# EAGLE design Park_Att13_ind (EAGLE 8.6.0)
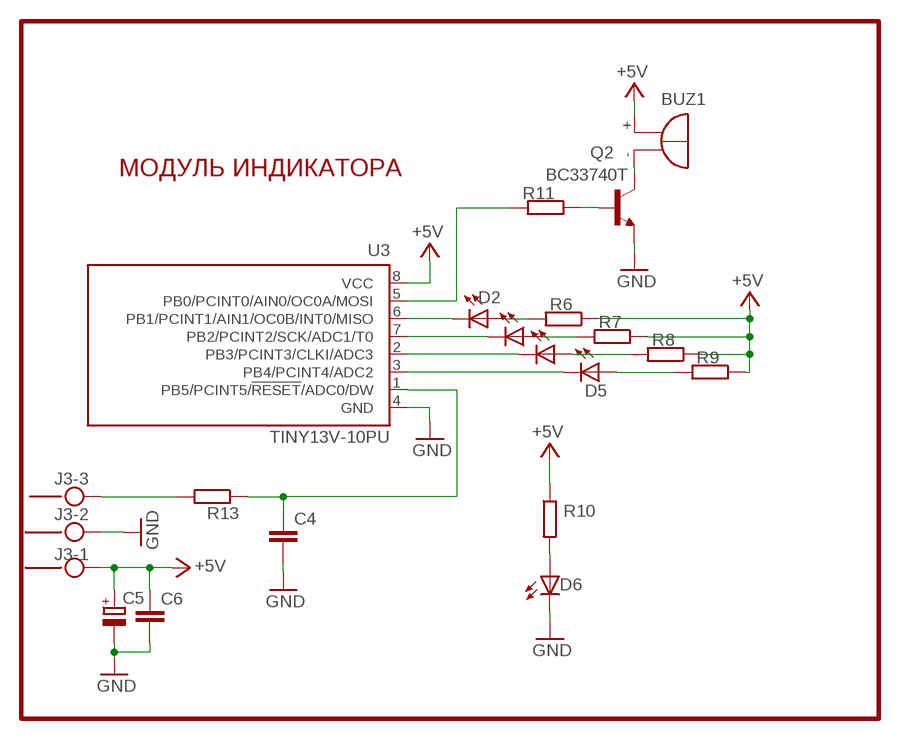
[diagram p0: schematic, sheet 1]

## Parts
BUZ1  F/HMB  [F/HMB]
C4  C-EUC1206  [C1206]
C5  CPOL-EUC/6032-28W  [C/6032-28W]
C6  C-EUC1206  [C1206]
D2  LED5MM  [LED5MM]
D3  LED5MM  [LED5MM]
D4  LED5MM  [LED5MM]
D5  LED5MM  [LED5MM]
D6  LED5MM  [LED5MM]
J3  MKDSN1,5/3-5,08  [MKDSN1,5/3-5,08]
Q2  BC33740T  BC337  [TO92]
R6  R-EU_R1206  [R1206]
R7  R-EU_R1206  [R1206]
R8  R-EU_R1206  [R1206]
R9  R-EU_R1206  [R1206]
R10  R-EU_R1206  [R1206]
R11  R-EU_R1206  [R1206]
R13  R-EU_R1206  [R1206]
U3  TINY13V-10PU  [DIL08]

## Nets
+5V: BUZ1.+ C5.+ C6.1 J3.1 R6.1 R7.1 R8.1 R9.1 R10.1 U3.8(VCC)
GND: C4.2 C5.- C6.2 D6.K(C) J3.2 Q2.1(E) U3.4(GND)
N$4: J3.3 R13.2
N$5: C4.1 R13.1 U3.1(PB5/PCINT5/!RESET!/ADC0/DW)
N$6: D2.K(C) U3.6(PB1/PCINT1/AIN1/OC0B/INT0/MISO)
N$7: D3.K(C) U3.7(PB2/PCINT2/SCK/ADC1/T0)
N$8: D4.K(C) U3.2(PB3/PCINT3/CLKI/ADC3)
N$9: D5.K(C) U3.3(PB4/PCINT4/ADC2)
N$10: R11.2 U3.5(PB0/PCINT0/AIN0/OC0A/MOSI)
N$11: D6.A R10.2
N$12: D3.A R7.2
N$13: D4.A R8.2
N$14: D5.A R9.2
N$17: D2.A R6.2
N$21: Q2.2(B) R11.1
N$22: BUZ1.- Q2.3(C)

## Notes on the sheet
- МОДУЛЬ ИНДИКАТОРА

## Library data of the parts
BUZ1 = buzzer:F/HMB: BUZZER; OC_FARNELL: unknown; OC_NEWARK: unknown
C4 C6 = rcl:C-EU: CAPACITOR, European symbol
C5 = rcl:CPOL-EU: POLARIZED CAPACITOR, European symbol
D2-D6 = led:LED: LED
J3 = con-phoenix-508:MKDSN1,5/3-5,08: MKDSN 1,5/ 3-5,08 Printklemme Nennstrom: 13,5 A Nennspannung: 250 V Rastermaß: 5,08 mm Polzahl: 3 Anschlussart: Schraubanschluss Montage: Löten Anschlussrichtung Leiter/Platine: 0 ° Artikelnummer: 1729131 Source: http://eshop.phoenixcontact.com .. 1729131.pdf
Q2 = transistor:BC337: NPN TRANSISTOR
R6-R11 R13 = rcl:R-EU_: RESISTOR, European symbol
U3 = atmel:TINY13: 8-bit AVR Microcontroller with 1K Bytes In-System Programmable Flash Source: http://www.atmel.com/dyn/resources/prod_documents/2535S.pdf; MPN: ATTINY13V-10PU; OC_FARNELL: 9171576; OC_NEWARK: 96K6523

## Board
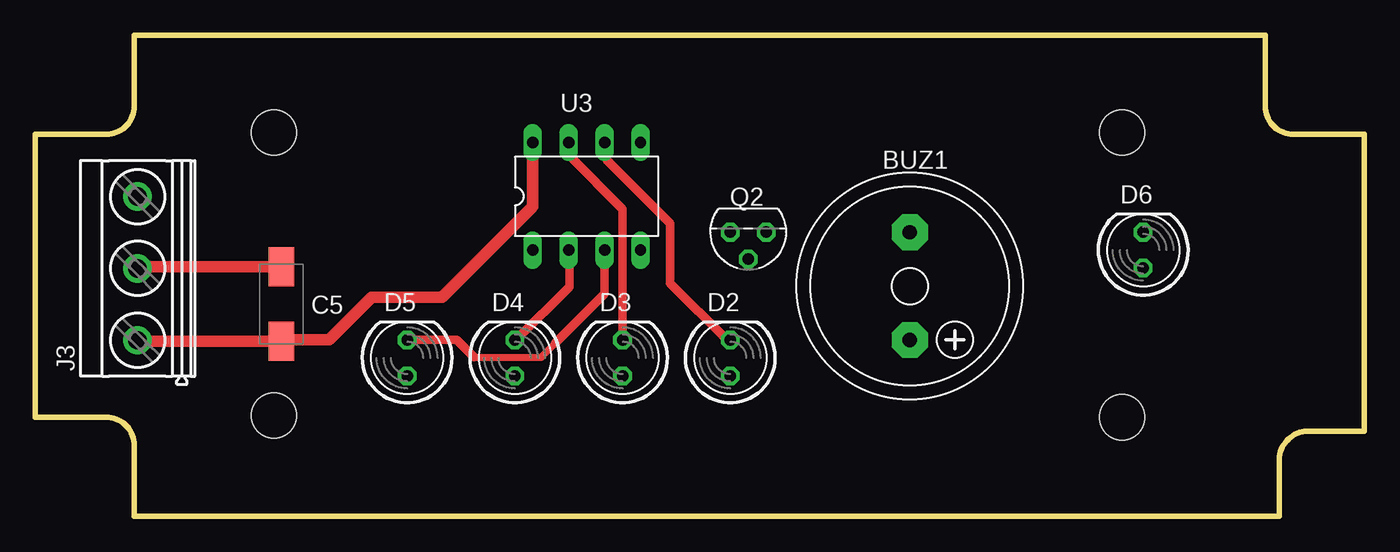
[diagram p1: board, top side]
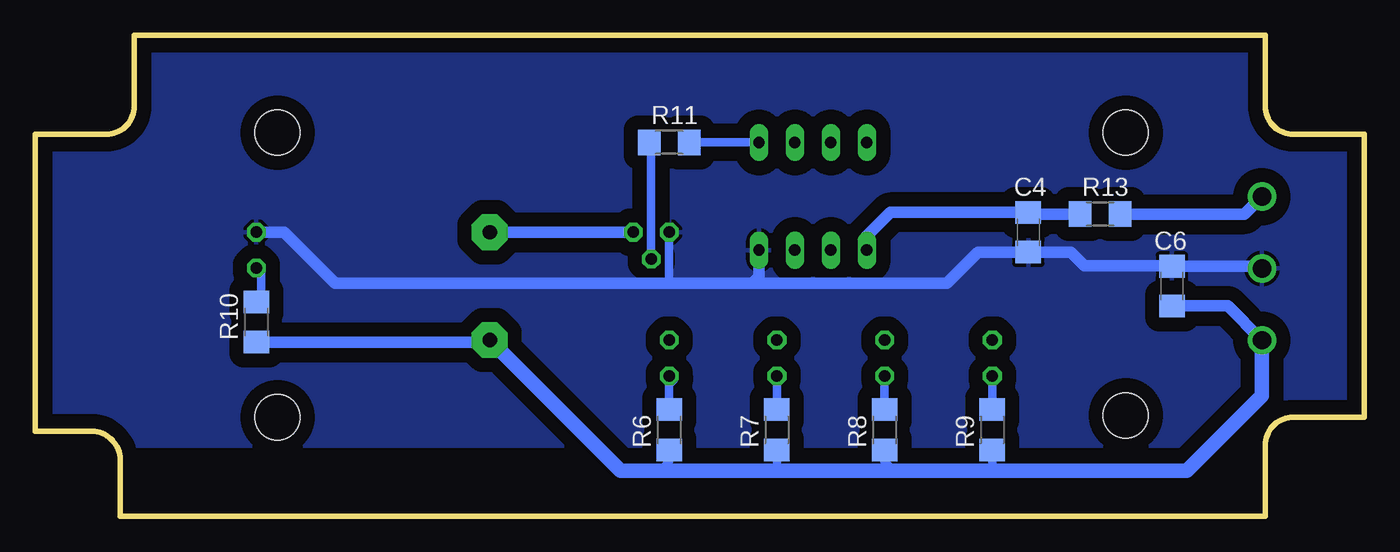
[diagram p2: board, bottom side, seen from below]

Size 94 x 34 mm. Coordinates in mm from the lower left corner, seen from the top.
Outline: 7,0 7,5 arc90 5,7 0,7 0,27 5,27 arc90 7,29 7,34 87,34 87,29 arc90 89,27 94,27 94,6 90,6 arc90 88,4 88,0 7,0
Copper layers (1*16): Top 0.035mm / dielectric 1.5mm / Bottom 0.035mm
Design rules "default": minimum track width 10mil, minimum drill 24mil, track to track 8mil, track to pad 8mil, pad to pad 8mil, via to via 8mil, smd to smd 8mil, copper to edge 40mil, drill to drill 8mil, minimum pad ring 10mil, minimum via ring 8mil, stop-mask expansion 4mil, vias tented up to drill 0mil, thermal gap 10mil
Holes 3.2 mm at 16.88,7.12 76.88,7 16.88,27.12 76.88,27.12

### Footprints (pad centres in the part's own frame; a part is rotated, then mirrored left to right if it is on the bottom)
F/HMB = drill 1.016 pad 2.54 octagon: + 3.81,0; - -3.81,0
C1206 = smd 1.6 x 1.8: 1 -1.4,0; 2 1.4,0
C/6032-28W = smd 2.75 x 1.8: + 2.625,0; - -2.625,0
LED5MM = drill 0.813 octagon: A -1.27,0; K 1.27,0
MKDSN1,5/3-5,08 = drill 1.3 pad 2: 1 -7.641,0.025; 2 -2.561,0.025; 3 2.519,0.025
TO92 = drill 0.813 octagon: 1 1.27,0; 2 0,1.905; 3 -1.27,0
R1206 = smd 1.6 x 1.803: 1 -1.422,0; 2 1.422,0
DIL08 = drill 0.813 long: 1 -3.81,-3.81; 2 -1.27,-3.81; 3 1.27,-3.81; 4 3.81,-3.81; 5 3.81,3.81; 6 1.27,3.81; 7 -1.27,3.81; 8 -3.81,3.81

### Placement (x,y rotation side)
BUZ1  61.86,16.27 270 top
C4  23.76,20.08 270 bottom
C5  17.41,15 270 top
C6  13.6,16.27 90 bottom
D2  49.16,11.19 90 top
D3  41.54,11.19 90 top
D4  33.92,11.19 90 top
D5  26.3,11.19 90 top
D6  78.37,18.81 90 top
J3  7.25,20.08 90 top
Q2  50.43,20.08 180 top
R6  49.16,6.11 90 bottom
R7  41.54,6.11 90 bottom
R8  33.92,6.11 90 bottom
R9  26.3,6.11 90 bottom
R10  78.37,13.73 90 bottom
R11  49.16,26.43 0 bottom
R13  18.68,21.35 0 bottom
U3  39,22.62 0 top

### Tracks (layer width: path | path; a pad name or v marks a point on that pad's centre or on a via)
+5V
  Top 0.813: U3.8 35.19,21.88 28.78,15.47 23.78,15.47 20.78,12.47 17.51,12.47 C5.+ 7.29,12.38 J3.1
  Bottom 0.61: R9.1 26.3,3.45 26.53,3.22 | R8.1 33.92,3.86 33.28,3.22 | R7.1 41.54,3.48 41.28,3.22 | R6.1 49.16,3.84 49.78,3.22
  Bottom 0.813: C6.1 9.66,14.87 J3.1 | R10.1 62.01,12.31 BUZ1.+
  Bottom 1.016: J3.1 7.23,8.53 12.53,3.22 26.53,3.22 33.28,3.22 41.28,3.22 49.78,3.22 52.62,3.22 BUZ1.+
GND
  Top 0.813: C5.- 7.33,17.62 J3.2
  Bottom 0.61: Q2.1 49.16,16.59 49.28,16.47
  Bottom 0.813: J3.2 7.38,17.67 C6.2 13.65,17.72 19.78,17.72 20.74,18.68 C4.2 27.32,18.68 29.53,16.47 43.28,16.47 | D6.K 76.39,20.08 72.78,16.47 49.28,16.47 43.28,16.47 | U3.4 42.81,16.94 43.28,16.47
  pour Bottom (isolate 1.016): 0.53,33.97 94.28,33.97 94.03,4.97 0.53,4.97
N$4
  Bottom 0.813: R13.2 8.47,21.35 J3.3
N$5
  Bottom 0.813: R13.1 23.63,21.35 C4.1 33.52,21.48 35.28,19.72 35.28,18.9 U3.1
N$6
  Top 0.61: D2.K 48.91,12.46 44.91,16.47 44.91,20.72 40.41,25.22 40.41,26.29 U3.6
N$7
  Top 0.61: D3.K 41.54,21.71 37.78,25.47 37.78,26.38 U3.7
N$8
  Top 0.61: D4.K 34.02,12.46 37.78,16.22 37.78,18.76 U3.2
N$9
  Top 0.5: 31.03,11.22 35.78,11.22 36.78,12.22
  Top 0.61: D5.K 29.79,12.46 31.03,11.22 | 36.78,12.22 40.28,15.72 U3.3
N$10
  Bottom 0.61: R11.2 U3.5
N$11
  Bottom 0.61: R10.2 78.35,15.15 78.03,15.47 78.03,17.2 D6.A
N$12
  Bottom 0.61: R7.2 D3.A
N$13
  Bottom 0.61: R8.2 D4.A
N$14
  Bottom 0.61: R9.2 D5.A
N$17
  Bottom 0.61: R6.2 49.16,9.34 48.78,9.72 48.96,9.72 D2.A
N$21
  Bottom 0.61: Q2.2 50.43,26.28 R11.1
N$22
  Bottom 0.813: BUZ1.- Q2.3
